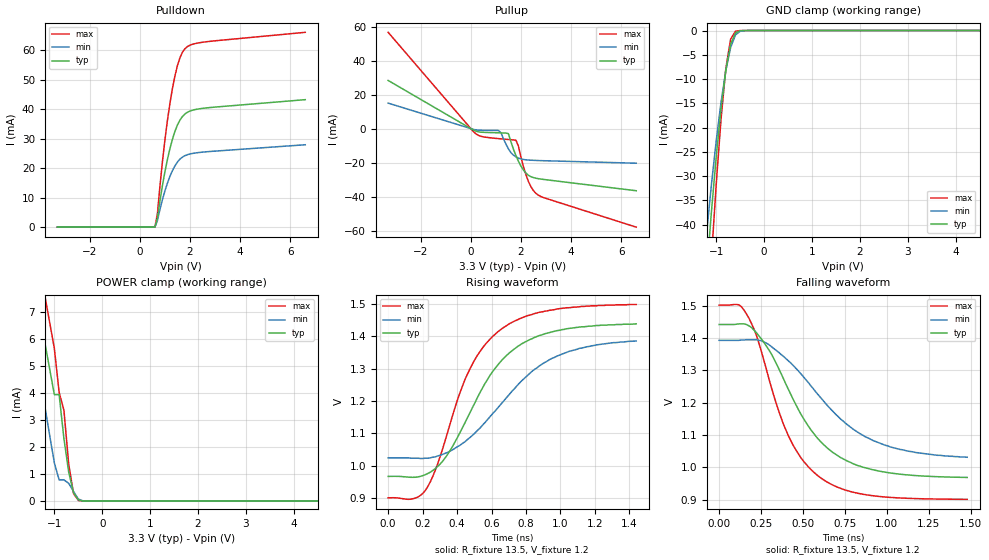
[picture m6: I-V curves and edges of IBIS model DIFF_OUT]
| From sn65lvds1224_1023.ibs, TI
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|   Model DIFF_OUT
| Developed by Mohamed Korany
[Model]   DIFF_OUT
Model_type   3-state
Polarity   Non-Inverting
Enable   Active-High
| Cref,Rref are extracted from datasheet , Vmeas , vref and C_comp
| measured by ICX. Vmeas and Vref is extracted using shunt resistance
| between the diffrential o/p equal 27 ohm
Vmeas = 1.21125V
Cref  = 10pF
Rref  = 13.5
Vref  = 1.21125V
| Ccomp are measured by ICX.
C_comp   17.51206pF   17.51206pF   17.51206pF
[Temperature Range]   27   85   -40
[Voltage Range]   3.3V   3.0V   3.6V
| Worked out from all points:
|   slope of the pullup table from 0 to 0.495 V, typ, clamps not added: 228 ohm
|   GND clamp passes 1 mA (typ) near -0.62 V on its own axis
|   POWER clamp passes 1 mA (typ) near -0.69 V on its own axis
|   rising waveform, R_fixture 13.5, V_fixture 1.2: 20-80 % time 319ps typ, 397ps min, 273ps max; typ from 0.966 V to 1.44 V
|   falling waveform, R_fixture 13.5, V_fixture 1.2: 20-80 % time 323ps typ, 411ps min, 262ps max; typ from 1.44 V to 0.968 V
[Pulldown]
| voltage   I(typ)   I(min)   I(max)
-3.3V     -424.1nA   -444.9nA   -408.9nA
600mV     141.4nA    130.3nA    156.6nA
700mV     3.043mA    2.248mA    4.583mA
800mV     8.858mA    5.981mA    13.87mA
1V        18.81mA    12.33mA    29.64mA
1.1V      22.99mA    14.96mA    36.23mA
1.3V      29.85mA    19.2mA     47.07mA
1.5V      34.7mA     22.11mA    54.85mA
1.6V      36.35mA    23.09mA    57.5mA
1.9V      39mA       24.59mA    61.29mA
2.7V      40.5mA     25.61mA    62.96mA
6.6V      43.26mA    27.96mA    66.11mA
[Pullup]
| voltage   I(typ)   I(min)   I(max)
-3.3V     28.31mA    14.98mA    56.61mA
200mV     -1.495mA   -752.7uA   -3.044mA
1.1V      -2.468mA   -1.094mA   -5.888mA
1.2V      -2.512mA   -2.425mA   -6.022mA
1.5V      -2.966mA   -11.9mA    -6.398mA
1.8V      -15.93mA   -16.61mA   -6.804mA
1.9V      -19.27mA   -17.31mA   -10.35mA
2.2V      -26.2mA    -18.36mA   -27.23mA
2.4V      -28.3mA    -18.58mA   -34.22mA
2.6V      -29.18mA   -18.72mA   -38.1mA
2.9V      -29.89mA   -18.88mA   -40.57mA
6.6V      -36.54mA   -20.35mA   -57.95mA
[GND_clamp]
| voltage   I(typ)   I(min)   I(max)
-3.3V     -394.4mA   -327mA     -489.1mA
-1.2V     -49.68mA   -41.63mA   -63.61mA
-1.1V     -37.19mA   -31.64mA   -46.82mA
-1V       -25.9mA    -22.63mA   -31.47mA
-900mV    -16.09mA   -14.75mA   -18.15mA
-800mV    -8.169mA   -8.232mA   -7.773mA
-700mV    -2.815mA   -3.485mA   -1.764mA
-600mV    -496.2uA   -922.9uA   -146.2uA
-500mV    -44.89uA   -140.1uA   -5.169uA
-300mV    -358.7nA   -1.368uA   -287.6nA
6.6V      335.7nA    1.048uA    316.3nA
[POWER_clamp]
| voltage   I(typ)   I(min)   I(max)
-3.3V     67.74mA    50.65mA    84.14mA
-1.6V     11.98mA    8.634mA    15.25mA
-1.5V     9.807mA    7.06mA     12.3mA
-1.4V     7.806mA    5.624mA    9.576mA
-1V       3.934mA    1.409mA    5.64mA
-900mV    3.934mA    785.2uA    4.017mA
-800mV    2.309mA    785.2uA    3.358mA
-700mV    1.066mA    657uA      1.359mA
-600mV    313.5uA    358.3uA    283.7uA
-500mV    46.14uA    77.67uA    25.84uA
-300mV    545nA      1.049uA    439.5nA
6.6V      0A         0A         0A
[Ramp]
| variable   typ   min   max
dV/dt_r 0.2835V/0.318857ns  0.2172V/0.397111ns  0.35934V/0.273262ns
dV/dt_f 0.2841V/0.322654ns  0.2172V/0.410626ns  0.36078V/0.261569ns
R_load = 13.5
[Rising Waveform]
R_fixture = 13.5
V_fixture = 1.2
V_fixture_min = 1.2
V_fixture_max = 1.2
| time   V(typ)   V(min)   V(max)
0s        966.5mV    1.024V     900.1mV
144ps     963.7mV    1.023V     897.3mV
216ps     971.9mV    1.023V     923.2mV
331.2ps   1.024V     1.038V     1.078V
460.8ps   1.149V     1.081V     1.284V
547.2ps   1.24V      1.125V     1.364V
662.4ps   1.328V     1.195V     1.425V
777.6ps   1.378V     1.264V     1.458V
950.4ps   1.414V     1.332V     1.482V
1.44ns    1.439V     1.386V     1.499V
[Falling Waveform]
R_fixture = 13.5
V_fixture = 1.2
V_fixture_min = 1.2
V_fixture_max = 1.2
| time   V(typ)   V(min)   V(max)
0s        1.442V     1.393V     1.502V
118.4ps   1.444V     1.393V     1.503V
177.6ps   1.438V     1.395V     1.462V
222ps     1.417V     1.395V     1.409V
310.8ps   1.352V     1.374V     1.249V
414.4ps   1.24V      1.329V     1.096V
592ps     1.087V     1.224V     972.7mV
725.2ps   1.03V      1.149V     934.5mV
917.6ps   992.3mV    1.083V     911.8mV
1.48ns    968.5mV    1.031V     900.7mV
